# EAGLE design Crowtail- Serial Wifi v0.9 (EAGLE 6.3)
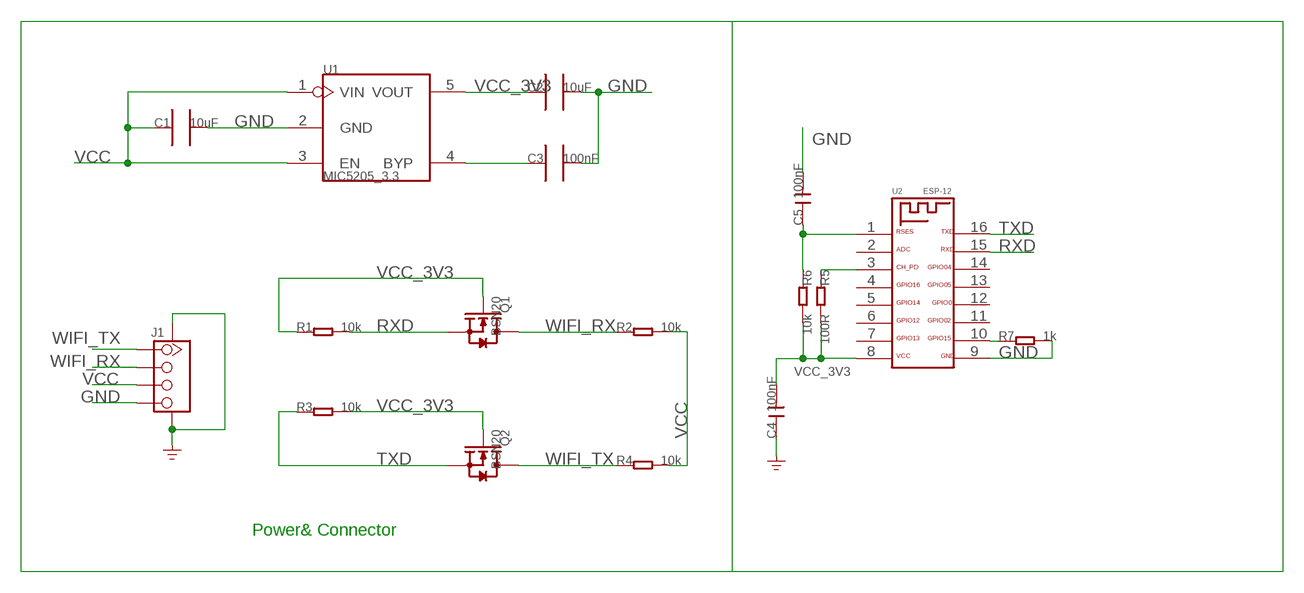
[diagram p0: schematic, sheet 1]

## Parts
C1  10uF  C0805_S  [0805_S]
C2  10uF  C0805_S  [0805_S]
C3  100nF  C0603_S  [0603_S]
C4  100nF  C-0603  [C0603]
C5  100nF  C-0603  [C0603]
J1  TWIG-4P-2.0-SMD-FEMALE-REINFORCE'90D'  [4P-SMD-2.0-90D]
Q1  BSN20  MOSFET-N'SOT23'  [SOT23]
Q2  BSN20  MOSFET-N'SOT23'  [SOT23]
R1  10k  R-0603  [R0603]
R2  10k  R-0603  [R0603]
R3  10k  R-0603  [R0603]
R4  10k  R-0603  [R0603]
R5  100R  R-0603  [R0603]
R6  10k  R-0603  [R0603]
R7  1k  R-0603  [R0603]
U1  MIC5205_3.3  MIC5025_X.X  [SOT23-5]
U2  ESP-12  [ESP-12]

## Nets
GND: C1.2 C2.2 C3.2 C4.1 C5.2 J1.4 J1.SS1 J1.SS2 R7.2 U1.2(GND) U2.9
N$2: R7.1 U2.10
N$3: C3.1 U1.4(BYP)
N$5: R5.1 U2.3
N$6: C5.1 R6.1 U2.1
RXD: Q1.2(S) R1.2 U2.15
TXD: Q2.2(S) R3.1 U2.16
VCC: C1.1 J1.3 R2.2 R4.2 U1.1(VIN) U1.3(EN)
VCC_3V3: C2.1 C4.2 Q1.1(G) Q2.1(G) R1.1 R3.2 R5.2 R6.2 U1.5(VOUT) U2.8
WIFI_RX: J1.2 Q1.3(D) R2.1
WIFI_TX: J1.1 Q2.3(D) R4.1
Unconnected: U2.2 U2.4 U2.5 U2.6 U2.7 U2.11 U2.12 U2.13 U2.14

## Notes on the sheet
- Power& Connector

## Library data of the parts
C1 C2 = CPT_SMD:C0805
C3 = CPT_SMD:C0603
C4 C5 = Discrete:C*: Ceramic Capacitors
J1 = Connector:TWIG-4P-2.0-SMD-FEMALE-REINFORCE
Q1 Q2 = Discrete:MOSFET-N: IRLL014: http://www.vishay.com/docs/91319/sihll014.pdf
R1-R7 = Discrete:R*
U1 = ICs_v54:MIC5025_X.X
U2 = Discrete:ESP-12

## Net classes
0 default: width 0.203 mm, drill 0.305 mm, clearance 0.203 mm

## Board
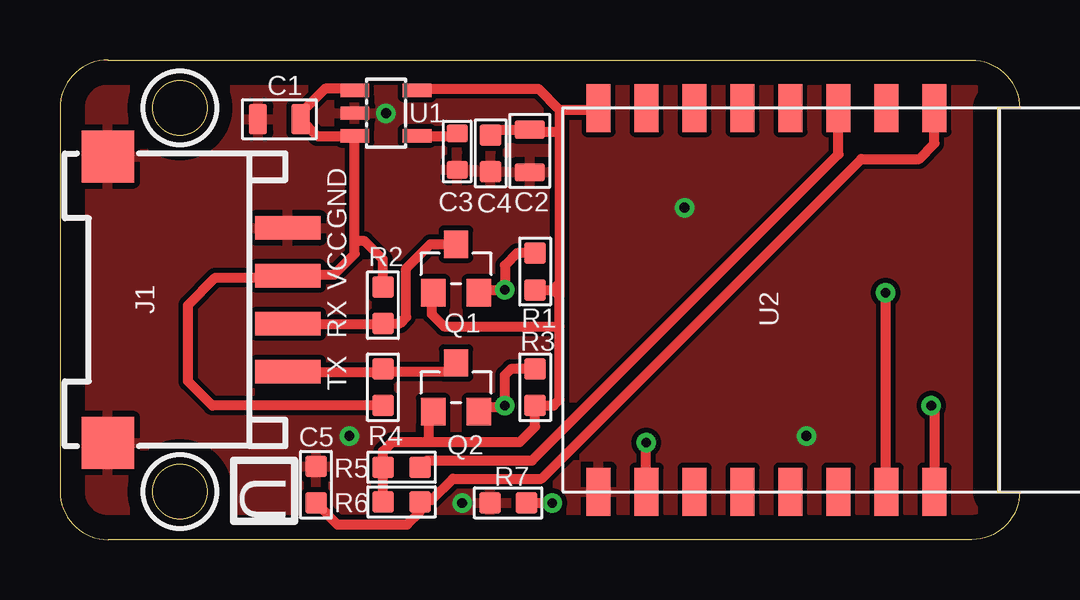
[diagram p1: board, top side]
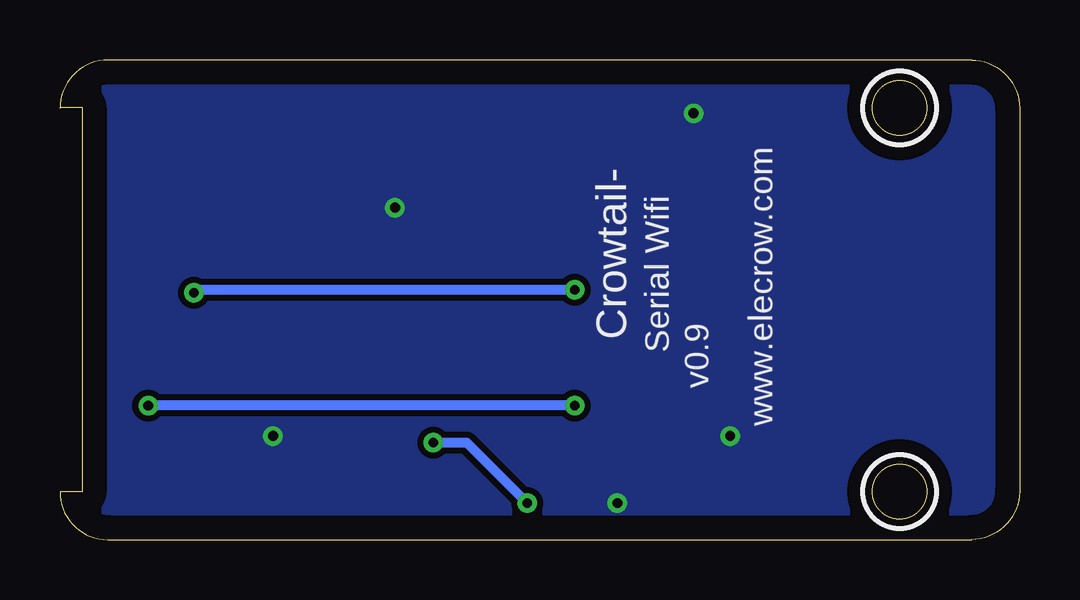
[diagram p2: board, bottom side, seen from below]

Size 40 x 20 mm. Coordinates in mm from the lower left corner, seen from the top.
Outline: 2,20 38,20 arc-90 40,18 40,18.02 39.08,18.02 39.08,1.98 40,1.98 arc-90 38.02,0 2,0 arc-90 0,2 0,18 arc-90 2,20
Outline: circle at 5,18 radius 1.14
Outline: circle at 5,2 radius 1.14
Copper layers (1*16): Top 0.035mm / dielectric 1.5mm / Bottom 0.035mm
Design rules "default *": minimum track width 10mil, minimum drill 24mil, track to track 8mil, track to pad 8mil, pad to pad 8mil, via to via 8mil, smd to smd 8mil, copper to edge 40mil, drill to drill 8mil, minimum pad ring 10mil, minimum via ring 8mil, stop-mask expansion 2mil, vias tented up to drill 100mil, thermal gap 10mil
tRestrict: area 3.5,16.5 to 6.5,19.5; area 3.5,0.5 to 6.5,3.5
bRestrict: area 3.5,16.5 to 6.5,19.5; area 3.5,0.5 to 6.5,3.5

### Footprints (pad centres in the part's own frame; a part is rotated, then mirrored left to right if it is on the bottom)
0805_S = smd 0.762 x 1.27: 1 -0.889,0; 2 0.889,0
0603_S = smd 0.762 x 0.889: 1 -0.762,0; 2 0.762,0
C0603 = smd 0.889 x 0.889: 1 -0.762,0; 2 0.762,0
4P-SMD-2.0-90D = smd 0.965 x 2.74: 1 -3,-0.1; 2 -1,-0.1; 3 1,-0.1; 4 3,-0.1 | smd 2.159 x 2.184: SS1 -5.974,7.4; SS2 5.974,7.4
SOT23 = smd 1.016 x 1.143: 1 -0.95,-1.016; 2 0.95,-1.016; 3 0,1.016
R0603 = smd 0.889 x 0.889: 1 -0.762,0; 2 0.762,0
SOT23-5 = smd 0.55 x 1.2: 1 -0.95,-1.3; 2 0,-1.3; 3 0.95,-1.3; 4 0.95,1.3; 5 -0.95,1.3
ESP-12 = smd 2 x 1: 1 0,15.5; 2 0,13.5; 3 0,11.5; 4 0,9.5; 5 0,7.5; 6 0,5.5; 7 0,3.5; 8 0,1.5; 9 16,1.5; 10 16,3.5; 11 16,5.5; 12 16,7.5; 13 16,9.5; 14 16,11.5; 15 16,13.5; 16 16,15.5

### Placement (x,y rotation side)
C1  9.14,17.53 180 top
C2  19.58,16.21 270 top
C3  16.56,16.18 270 top
C4  17.96,16.1 90 top
C5  10.67,2.29 90 top
J1  9.4,10 90 top
Q1  16.51,11.3 0 top
Q2  16.51,6.35 0 top
R1  19.81,11.18 90 top
R2  13.46,9.78 90 top
R3  19.81,6.35 270 top
R4  13.46,6.35 270 top
R5  14.24,3.02 180 top
R6  14.24,1.57 180 top
R7  18.68,1.52 180 top
U1  13.59,17.78 270 top
U2  20.95,18 270 top

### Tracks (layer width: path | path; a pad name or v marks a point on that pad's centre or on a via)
GND  (via drill 0.41)
  other vias: 12.06,4.32 31.11,4.32 16.76,1.52 26.04,13.84 13.59,17.78
  pour Top: -1.27,20.32 41.91,20.32 41.91,0.05 arc-90 41.86,0 -1.27,0
  pour Bottom (isolate 0.254): -1.27,20.32 41.91,20.32 41.91,0 -1.27,0
N$2  (via drill 0.41)
  Top 0.406: R7.1 v20.52,1.52 | U2.10 24.43,2 v24.43,4.04
  Bottom 0.406: v20.52,1.52 23.04,4.04 v24.43,4.04
N$3
  Top 0.406: U1.4 16.56,16.83 C3.1
N$5
  Top 0.406: U2.3 32.45,16.07 19.68,3.3 15.29,3.3 R5.1
N$6
  Top 0.406: R6.1 14.92,1.52 | 36.58,18.54 36.45,18.42 U2.1 36.45,16.52 35.81,15.88 33.4,15.88 20.07,2.54 16.38,2.54 15.49,1.65 15.08,1.65 R6.1 | C5.1 11.56,0.64 14.48,0.64 15,1.16 R6.1
RXD  (via drill 0.41)
  Top 0.406: R1.2 19.05,11.94 18.54,11.43 v18.54,10.41 17.46,10.41 Q1.2 | U2.15 34.42,2.07 v34.42,10.29
  Bottom 0.406: v18.54,10.41 34.42,10.41 v34.42,10.29
TXD  (via drill 0.41)
  Top 0.406: 17.53,5.33 Q2.2 17.46,5.52 18.22,5.52 18.29,5.59 v18.54,5.59 18.54,6.86 18.8,7.11 R3.1 | v36.32,5.59 36.45,5.46 U2.16
  Bottom 0.406: v18.54,5.59 v36.32,5.59
VCC
  Top 0.406: R4.2 6.35,5.59 5.33,6.6 5.33,9.78 6.48,10.92 9.42,10.92 J1.3 10.62,11 10.67,11.05 11.43,11.05 12.29,11.91 12.29,12.45 | U1.3 10.73,16.83 C1.1 10.03,17.78 11.05,18.8 12.22,18.8 U1.1 | U1.3 12.32,16.8 | 12.29,12.45 U1.3 | R2.2 13.46,11.68 12.7,12.45 12.29,12.45
VCC_3V3
  Top 0.406: 20.83,17.91 20.83,17.02 | 20.83,17.02 20.83,10.67 | 20.83,10.67 20.83,10.16 | R1.1 20.57,10.41 | 20.57,10.41 20.83,10.16 | 20.83,10.67 20.57,10.41 | 22.48,18.01 U2.8 22.36,17.91 20.83,17.91 | U1.5 14.95,18.67 15.08,18.8 19.94,18.8 20.83,17.91 | 15.37,4.06 13.84,4.06 13.46,3.68 13.46,3.13 R5.2 R6.2 | 15.37,4.06 19.18,4.06 19.81,4.7 R3.2 20.57,5.59 20.83,5.84 20.83,8.89 | 20.83,8.89 20.83,10.16 | Q2.1 15.37,5.14 15.37,4.06 | 20.83,17.02 19.66,17.02 C2.1 18.19,17.09 C4.2 | Q1.1 15.49,10.22 15.49,9.4 16,8.89 20.83,8.89
WIFI_RX
  Top 0.406: 9.52,9.02 J1.2 13.46,9 R2.1 14.17,9.02 14.43,9.27 14.43,11.3 15.44,12.32 Q1.3
WIFI_TX
  Top 0.406: 9.5,7.11 J1.1 13.46,7 R4.1 13.56,7.01 16.08,7.01 16.43,7.37 Q2.3

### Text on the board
tPlace: GND | VCC | RX | TX | U
bPlace: www.elecrow.com | Crowtail- | Serial Wifi | v0.9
